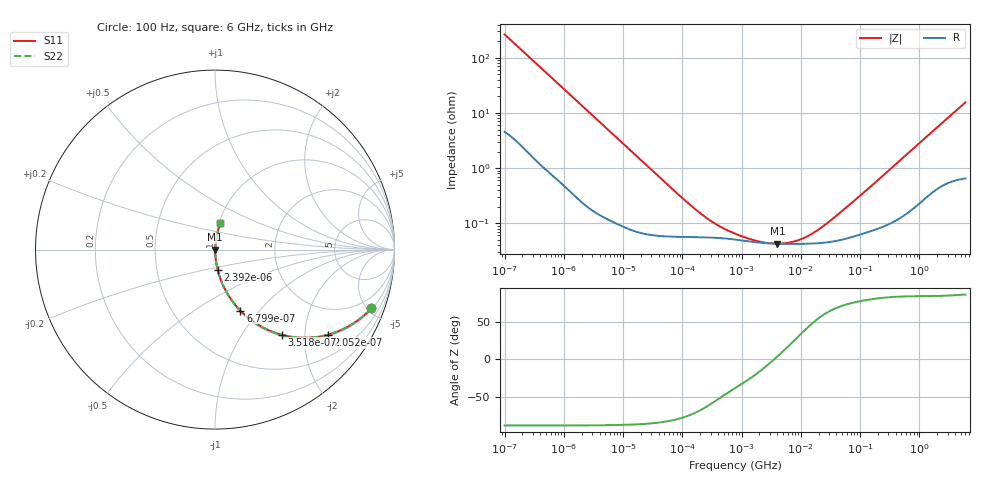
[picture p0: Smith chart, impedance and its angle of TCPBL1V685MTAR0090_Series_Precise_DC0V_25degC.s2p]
! TCPBL1V685MTAR0090 Polymer Tantalum Capacitor Sparameter Model
! Model Generated by Samsung Electro-Mechanics
! Samsung Sparameter Version 5.0
! Date : Oct-10-2024
! Products : Polymer Tantalum Capacitor
! Characteristics :
!  Nominal Capacitance = 6.8uF
!  Capacitance Tolerance = +/-20%
!  ESR = 90 mohm max at 100kHz
!  Rated Voltage = 35Vdc
!  Size = 1411(unit:inch), 3528(unit:mm)
!  Length = 3.50+/-0.20mm
!  Width = 2.80+/-0.20mm
!  Thickness = 1.10+/-0.10mm
!  Lineup = Conductive Polymer Type
!  Feature = PBL
!  Measurement Temperature : 25degC.
!  DC bias Value = 0V
!  Frequency : 100Hz ~ 6GHz
! External Node Assignments :
!  1  o---||---o  2
# MHz S RI R 50.0
! Freq.  Real(S11)  Im(S11)  Real(S12)  Im(S12)  Real(S21)  Im(S21)  Real(S22)  Im(S22)
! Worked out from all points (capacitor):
!   300 points, 100 Hz to 6 GHz, reference 50 ohm
!   read as one part in series: C = 5.99 uF near 106.2 Hz
!   lowest |Z| = 42.7 mohm at 4.022 MHz (marker M1)
!   series resonance near 3.53 MHz, so ESL is about 340 pH
!   S11 on the Smith chart (normalised r, x): 100 Hz: 1.09, -5.30; 205.2 Hz: 1.05, -2.61; 351.8 Hz: 1.03, -1.53; 679.9 Hz: 1.01, -0.80; 2.392 kHz: 1.00, -0.23; 6 GHz: 1.01, +0.31
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0.0001  0.871 -0.3267  0.129 0.3267  0.129 0.3267  0.871 -0.3267
0.0001432463  0.7714 -0.4109  0.2286 0.4109  0.2286 0.4109  0.7714 -0.4109
0.0002051949  0.6276 -0.4745  0.3724 0.4745  0.3724 0.4745  0.6276 -0.4745
0.0003517965  0.3715 -0.4747  0.6285 0.4747  0.6285 0.4747  0.3715 -0.4747
0.0005039354  0.2272 -0.4105  0.7728 0.4105  0.7728 0.4105  0.2272 -0.4105
0.0006798988  0.1415 -0.3399  0.8585 0.3399  0.8585 0.3399  0.1415 -0.3399
0.001097881  0.0617 -0.2319  0.9383 0.2319  0.9383 0.2319  0.0617 -0.2319
0.001998454  0.0207 -0.134  0.9793 0.134  0.9793 0.134  0.0207 -0.134
0.00239186  0.015 -0.1128  0.985 0.1128  0.985 0.1128  0.015 -0.1128
0.007030492  0.00257 -0.0392  0.9974 0.0392  0.9974 0.0392  0.00257 -0.0392
0.03993819  0.000639 -0.007  0.9994 0.007  0.9994 0.007  0.000639 -0.007
0.2408823  0.000556 -0.00119  0.9994 0.00119  0.9994 0.00119  0.000556 -0.00119
0.4384739  0.000539 -0.000676  0.9995 0.000676  0.9995 0.000676  0.000539 -0.000676
0.7981464  0.000505 -0.000395  0.9995 0.000395  0.9995 0.000395  0.000505 -0.000395
1.960157  0.000446 -0.000136  0.9996 0.000136  0.9996 0.000136  0.000446 -0.000136
4.022142  0.000426 3.01e-05  0.9996 -3.01e-05  0.9996 -3.01e-05  0.000426 3.01e-05
8.253232  0.000422 0.000222  0.9996 -0.000222  0.9996 -0.000222  0.000422 0.000222
15.95059  0.000429 0.0005  0.9996 -0.0005  0.9996 -0.0005  0.000429 0.0005
41.59096  0.000484 0.00134  0.9995 -0.00134  0.9995 -0.00134  0.000484 0.00134
318.7652  0.00107 0.00937  0.9989 -0.00937  0.9989 -0.00937  0.00107 0.00937
1922.593  0.00674 0.0519  0.9933 -0.0519  0.9933 -0.0519  0.00674 0.0519
6000  0.0297 0.1502  0.9703 -0.1502  0.9703 -0.1502  0.0297 0.1502
